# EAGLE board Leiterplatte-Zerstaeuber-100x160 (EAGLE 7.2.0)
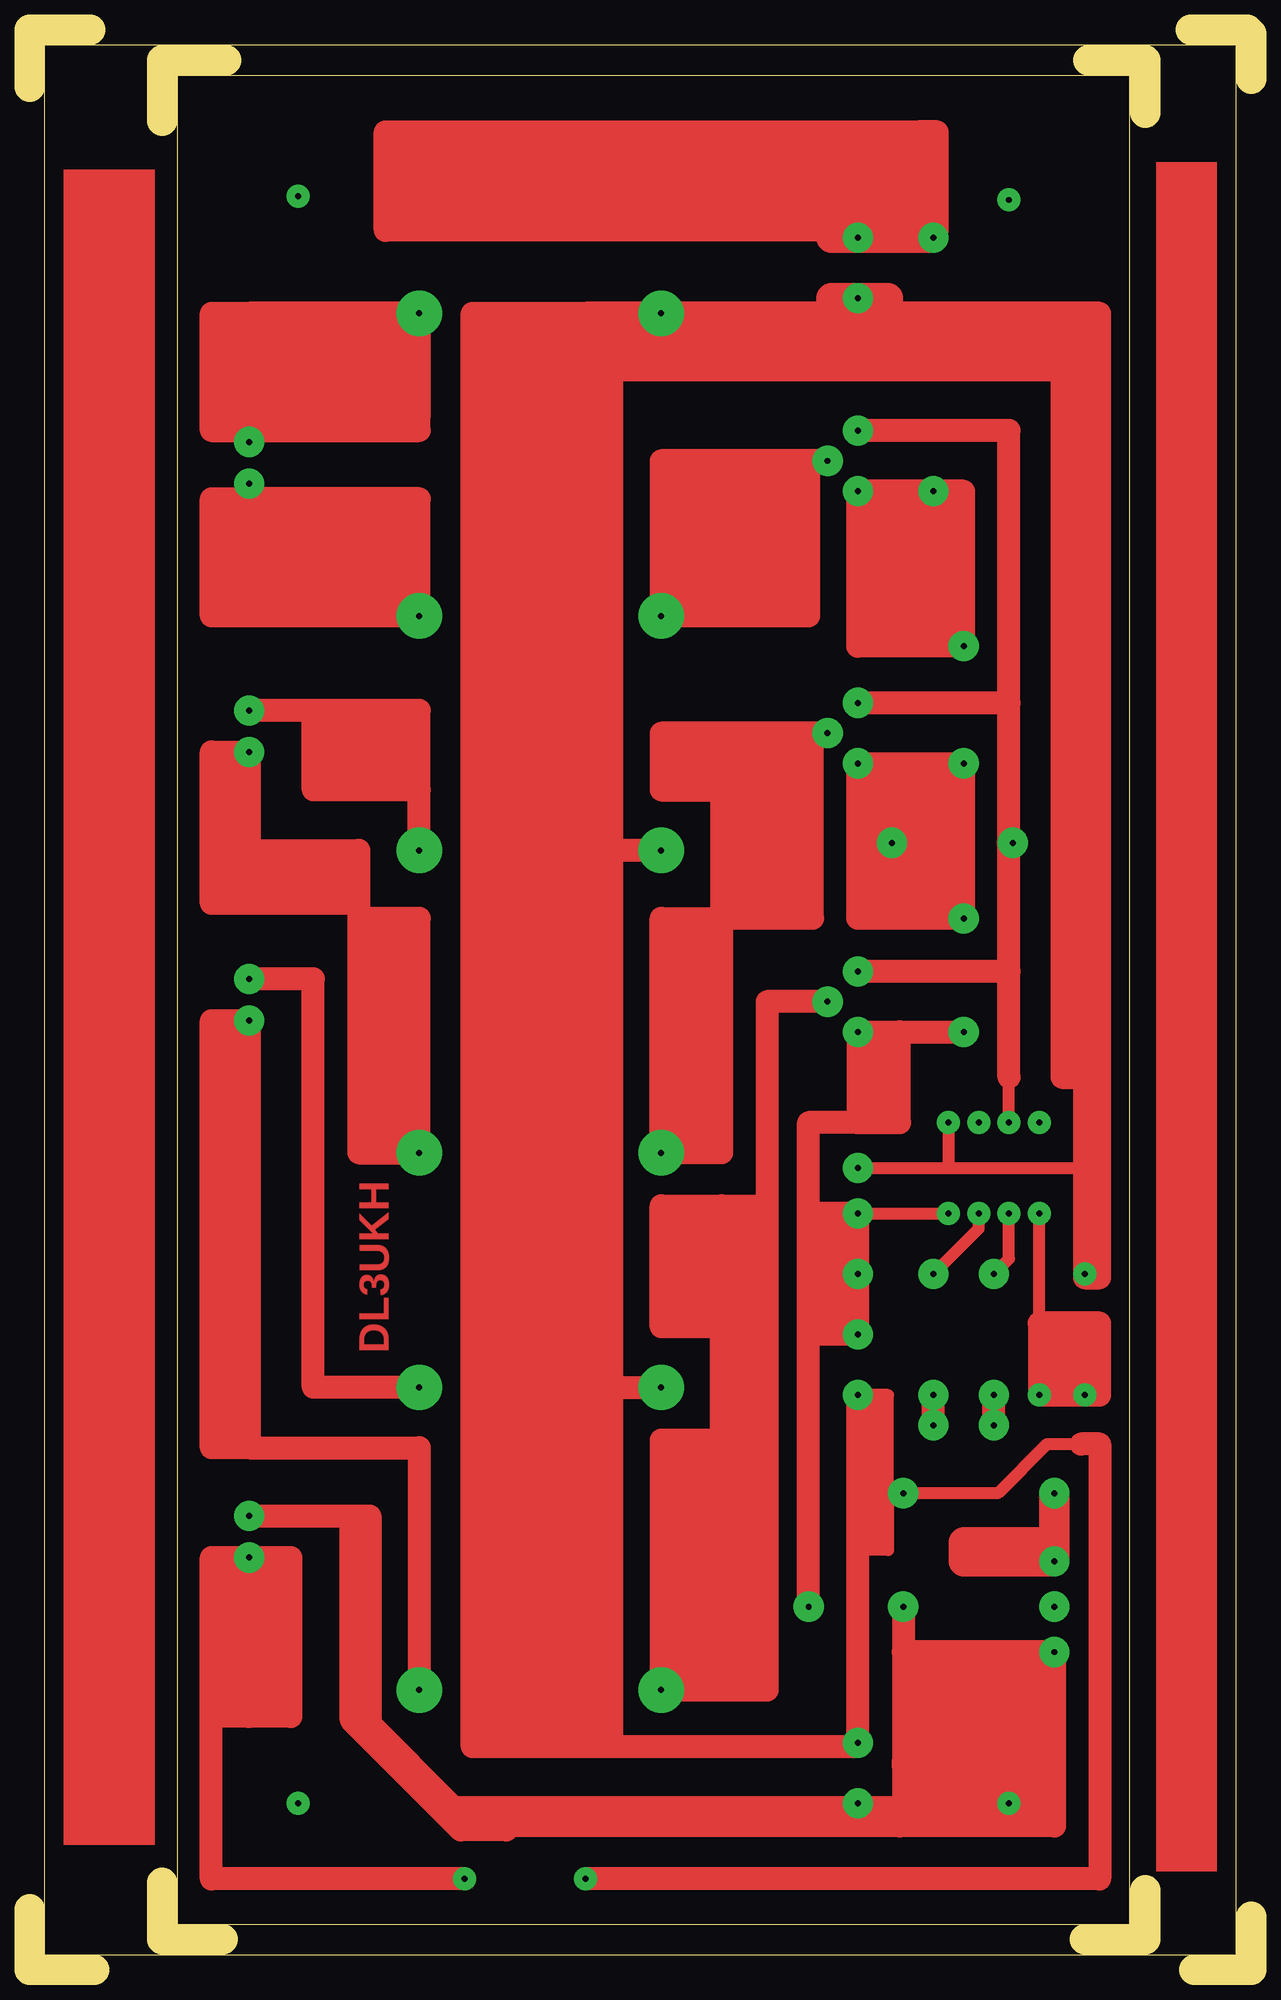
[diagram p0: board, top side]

Size 102.55 x 162.88 mm. Coordinates in mm from the lower left corner, seen from the top.
Outline: 5.4,0 0.32,0
Outline: 0,0 0,5.08
Outline: 97.79,0 102.55,0 102.55,4.45
Outline: 5.08,162.88 0,162.88 0,158.12
Outline: 102.55,158.75 102.55,162.56
Outline: 97.47,162.88 102.23,162.88
Outline: 16.51,160.34 11.43,160.34
Outline: 11.11,160.34 11.11,155.26
Outline: 88.9,160.34 93.66,160.34 93.66,155.89
Outline: 16.19,2.54 11.11,2.54 11.11,7.3
Outline: 93.66,6.67 93.66,2.54
Outline: 88.58,2.54 93.34,2.54
Outline: 1.27,1.27 101.28,1.27 101.28,161.61 1.27,161.61 1.27,1.27
Outline: 12.38,159.07 92.39,159.07 92.39,3.81 12.38,3.81 12.38,159.07
Copper layers (1*16): Top 0.035mm / dielectric 1.5mm / Bottom 0.035mm
Design rules "default": minimum track width 10mil, minimum drill 24mil, track to track 8mil, track to pad 8mil, pad to pad 8mil, via to via 8mil, smd to smd 8mil, copper to edge 40mil, drill to drill 8mil, minimum pad ring 10mil, minimum via ring 8mil, stop-mask expansion 4mil, vias tented up to drill 0mil, thermal gap 10mil

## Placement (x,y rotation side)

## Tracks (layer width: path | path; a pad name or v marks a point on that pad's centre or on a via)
S$1  (via drill 0.5 pad 1.93)
  other vias: 82.23,13.97
S$2  (via drill 0.5 pad 1.93)
  other vias: 22.54,13.97
S$3  (via drill 0.5 pad 1.93)
  other vias: 82.23,148.59
S$4  (via drill 0.5 pad 1.93)
  other vias: 22.54,148.91
S$5  (via drill 0.5 pad 1.93)
  other vias: 46.67,7.62
S$6  (via drill 0.5 pad 2.54)
  Top 1.016: 72.71,13.65 73.34,13.97 73.34,17.46
  Top 1.93: v18.41,38.1 28.57,38.1 28.57,20.64 35.56,13.65 72.71,13.65 73.34,13.65 | 73.34,30.48 73.34,26.67 | 73.34,26.67 73.34,13.97 | 86.04,17.46 v86.04,26.67 73.34,26.67 | 86.04,17.46 73.34,17.46 | 86.04,17.46 86.04,12.06 73.02,12.06 | 73.02,12.06 73.98,16.83 73.34,17.14 | 73.02,12.06 38.1,12.06
S$7  (via drill 0.5 pad 2.54)
  Top 1.016: v69.53,63.5 77.15,63.5 | 65.72,58.42 65.09,58.42 | 65.09,63.5 65.72,63.5 | 65.09,58.42 65.09,63.5 | 65.09,53.34 65.09,58.42 | 66.04,53.34 65.09,53.34 | 65.09,30.16 65.09,53.34 | 65.09,63.5 65.09,71.12 65.41,71.12
  Top 1.93: v69.53,58.42 65.72,58.42 | 66.04,53.34 v69.53,53.34 v69.53,63.5 65.72,63.5 | 73.02,78.74 v69.53,78.74 69.53,71.12 | 73.02,78.74 v78.42,78.74 | 69.53,71.12 65.41,71.12 v65.41,30.48 | 69.53,71.12 73.02,71.12 73.02,78.74
S$8  (via drill 0.5 pad 2.54)
  Top 1.93: v80.96,45.72 v80.96,48.26
S$9  (via drill 0.5 pad 2.54)
  Top 1.93: v75.88,45.72 v75.88,48.26
S$10  (via drill 0.5 pad 2.54, 0.5 pad 3.81)
  Top 1.93: v18.41,102.23 18.41,93.98 | 18.41,93.98 27.62,93.98 27.62,89.53 | 27.62,89.53 27.62,88.27 | 27.62,88.27 27.62,68.58 v32.7,68.58 32.7,88.27 27.62,88.27 | 18.41,93.98 15.24,93.98 | 15.24,93.98 15.24,102.23 18.1,102.23 | 27.62,89.53 15.24,89.53 15.24,93.98
S$11  (via drill 0.5 pad 2.54)
  Top 1.93: v78.42,88.27 69.53,88.27 v69.53,101.28 v78.42,101.28 v78.42,88.27
S$12  (via drill 0.5 pad 2.54, 0.5 pad 3.81)
  Top 1.93: v66.99,81.28 61.91,81.28 61.91,44.45 | 61.91,44.45 61.91,23.5 v53.02,23.5 53.02,44.45 58.1,44.45 | 61.91,44.45 58.1,44.45 | 58.1,44.45 58.1,53.98 | 58.1,53.98 58.1,64.14 | 58.1,64.14 61.6,64.14 | 58.1,53.98 53.02,53.98 53.02,64.14 58.1,64.14
S$13  (via drill 0.5 pad 2.54)
  Top 1.93: 86.04,35.56 86.04,35.88
  Top 2.54: v86.04,40.01 86.04,35.88 78.42,35.88 78.42,34.29 v86.04,34.29 86.04,35.56
S$14  (via drill 0.5 pad 2.54, 0.5 pad 3.81)
  Top 1.93: v32.7,48.9 23.81,48.9 23.81,83.19 v18.41,83.19
S$15  (via drill 0.5 pad 2.54)
  other vias: 73.34,30.48
S$16  (via drill 0.5 pad 2.54)
  Top 1.93: v78.42,111.12 69.53,111.12 v69.53,124.14 v75.88,124.14 78.42,124.14 v78.42,111.12
S$17  (via drill 0.5 pad 2.54, 0.5 pad 3.81)
  Top 1.93: 18.41,43.82 v18.41,79.69 15.24,79.69 15.24,43.82 18.41,43.82 | 18.41,43.82 32.7,43.82 v32.7,23.5
S$18  (via drill 0.5 pad 2.54, 0.5 pad 3.81)
  Top 1.93: v32.7,93.98 32.7,99.06 | 32.7,99.06 32.7,105.73 v18.41,105.73 | 32.7,99.06 23.81,99.06 23.81,105.41
S$19  (via drill 0.5 pad 2.54)
  other vias: 69.53,13.97
S$20  (via drill 0.5 pad 2.54)
  other vias: 86.04,30.48
S$21  (via drill 0.5 pad 1.93)
  Top 1.016: v88.58,48.26 88.58,54.61 84.77,54.61 | 84.77,54.61 v84.77,63.5 | 84.77,54.29 84.77,54.61
  Top 1.93: v88.58,48.26 89.85,48.26 89.85,54.29 84.77,54.29 v84.77,48.26 v88.58,48.26
S$22  (via drill 0.5 pad 2.54, 0.5 pad 3.81)
  Top 1.93: 18.41,139.06 v32.7,139.06 32.7,130.49 | 18.41,139.06 v18.41,128.27 | 15.24,129.22 15.24,139.06 18.41,139.06 | 32.7,130.49 17.78,130.49 | 32.7,129.22 32.7,130.49
S$23  (via drill 0.5 pad 1.93, 0.5 pad 2.54)
  Top 1.016: v80.96,58.42 82.23,59.69 v82.23,63.5
S$24  (via drill 0.5 pad 1.93, 0.5 pad 2.54)
  Top 1.93: v36.51,7.62 15.24,7.62 15.24,21.27 | 15.24,21.27 15.24,34.61 v18.41,34.61 | v18.41,34.61 18.41,21.27 | 18.41,21.27 15.24,21.27 | v18.41,34.61 21.91,34.61 21.91,21.27 18.41,21.27
S$25  (via drill 0.5 pad 2.54)
  other vias: 82.55,94.61
S$26  (via drill 0.5 pad 1.93, 0.5 pad 2.54)
  Top 1.016: v75.88,58.42 79.69,62.23 v79.69,63.5
S$27
  Top 1.93: 86.68,133.99 86.68,74.93 88.27,74.93
S$28  (via drill 0.5 pad 2.54)
  other vias: 72.39,94.61
S$29  (via drill 0.5 pad 2.54, 0.5 pad 3.81)
  Top 1.93: v66.99,126.68 65.41,126.68 | 65.41,126.68 53.02,126.68 v53.02,113.66 65.41,113.66 65.41,126.68
S$30
  Top 1.93: 40.01,11.75 36.2,11.75 26.99,20.95 26.99,37.78
S$31
  Top 1.93: 74.61,146.05 29.84,146.05 29.84,154.31 74.61,154.31 | 74.61,154.31 74.61,146.05 | 74.61,146.05 76.2,146.05 76.2,154.31 74.61,154.31
S$32  (via drill 0.5 pad 2.54, 0.5 pad 3.81)
  Top 1.93: v66.99,103.82 65.72,103.82 | 65.72,103.82 58.1,103.82 | 58.1,103.82 58.1,88.27 | 58.1,88.27 58.1,68.58 v53.02,68.58 53.02,88.27 58.1,88.27 | 58.1,88.27 65.72,88.27 65.72,103.82 | 58.1,103.82 53.02,103.82 53.02,99.06 57.47,99.06
S$33  (via drill 0.5 pad 1.93, 0.5 pad 2.54, 0.5 pad 3.81)
  Top 1.016: v77.15,71.12 77.15,67.31 | 77.15,67.31 88.58,67.31 | v69.53,67.31 77.15,67.31 | 88.27,44.13 85.41,44.13 81.28,40.01 v73.34,40.01 | v69.53,48.26 72.07,48.26 72.07,40.01 72.07,35.24 69.85,35.24
  Top 1.93: 88.58,58.1 89.85,58.1 89.85,139.06 88.58,139.06 | 88.58,134.3 88.58,67.31 v88.58,58.42 | 88.58,134.3 88.58,139.06 | 46.67,139.06 v53.02,139.06 88.58,139.06 | 46.67,139.06 46.67,134.3 | 46.67,134.3 46.67,93.98 | v53.02,93.98 46.67,93.98 | 46.67,93.98 46.67,48.9 | 46.67,48.9 v53.02,48.9 | 46.67,18.73 46.67,48.9 | 48.9,18.73 69.53,18.73 v69.53,19.05 69.53,40.01 | 48.9,18.73 46.67,18.73 | 88.58,134.3 46.67,134.3 | 48.9,18.73 48.9,135.57 49.21,135.57 | 46.67,18.73 37.15,18.73 37.15,139.06 46.67,139.06 | 46.67,7.62 89.85,7.62 89.85,44.13 88.27,44.13 | 69.53,40.01 v69.53,48.26 | v73.34,40.01 72.07,40.01 69.53,40.01
S$34  (via drill 0.5 pad 2.54)
  Top 2.54: v69.53,140.34 69.53,138.11 | 72.07,138.43 72.07,140.34 v69.53,140.34 | v69.53,140.34 67.31,140.34 67.31,137.48
S$35  (via drill 0.5 pad 1.93)
  other vias: 77.15,63.5
S$36  (via drill 0.5 pad 2.54)
  Top 2.54: 75.88,145.42 v69.53,145.42 67.31,145.42
S$38  (via drill 0.5 pad 2.54, 0.5 pad 3.81)
  Top 1.93: 32.7,123.51 v32.7,113.66 18.41,113.66 | 18.41,113.66 v18.41,124.78 | 18.41,113.66 15.24,113.66 15.24,122.87 | 15.24,122.87 18.73,122.87 | 15.24,122.87 15.24,123.51 18.73,123.51
S$39  (via drill 0.5 pad 1.93)
  other vias: 79.69,71.12
S$40  (via drill 0.5 pad 2.54)
  other vias: 75.88,145.42
S$49  (via drill 0.5 pad 1.93, 0.5 pad 2.54)
  Top 1.016: v82.23,71.12 82.23,74.93
  Top 1.93: 82.23,83.82 v69.53,83.82 | 82.23,83.82 82.23,106.36 | 82.23,106.36 v69.53,106.36 | 82.23,106.36 82.23,129.22 v69.53,129.22 | 82.23,74.93 82.23,83.82
S$56  (via drill 0.5 pad 1.93)
  other vias: 84.77,71.12
(copper drawn outside any net)
  shapes: Top area x34

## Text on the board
Top: DL3UKH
